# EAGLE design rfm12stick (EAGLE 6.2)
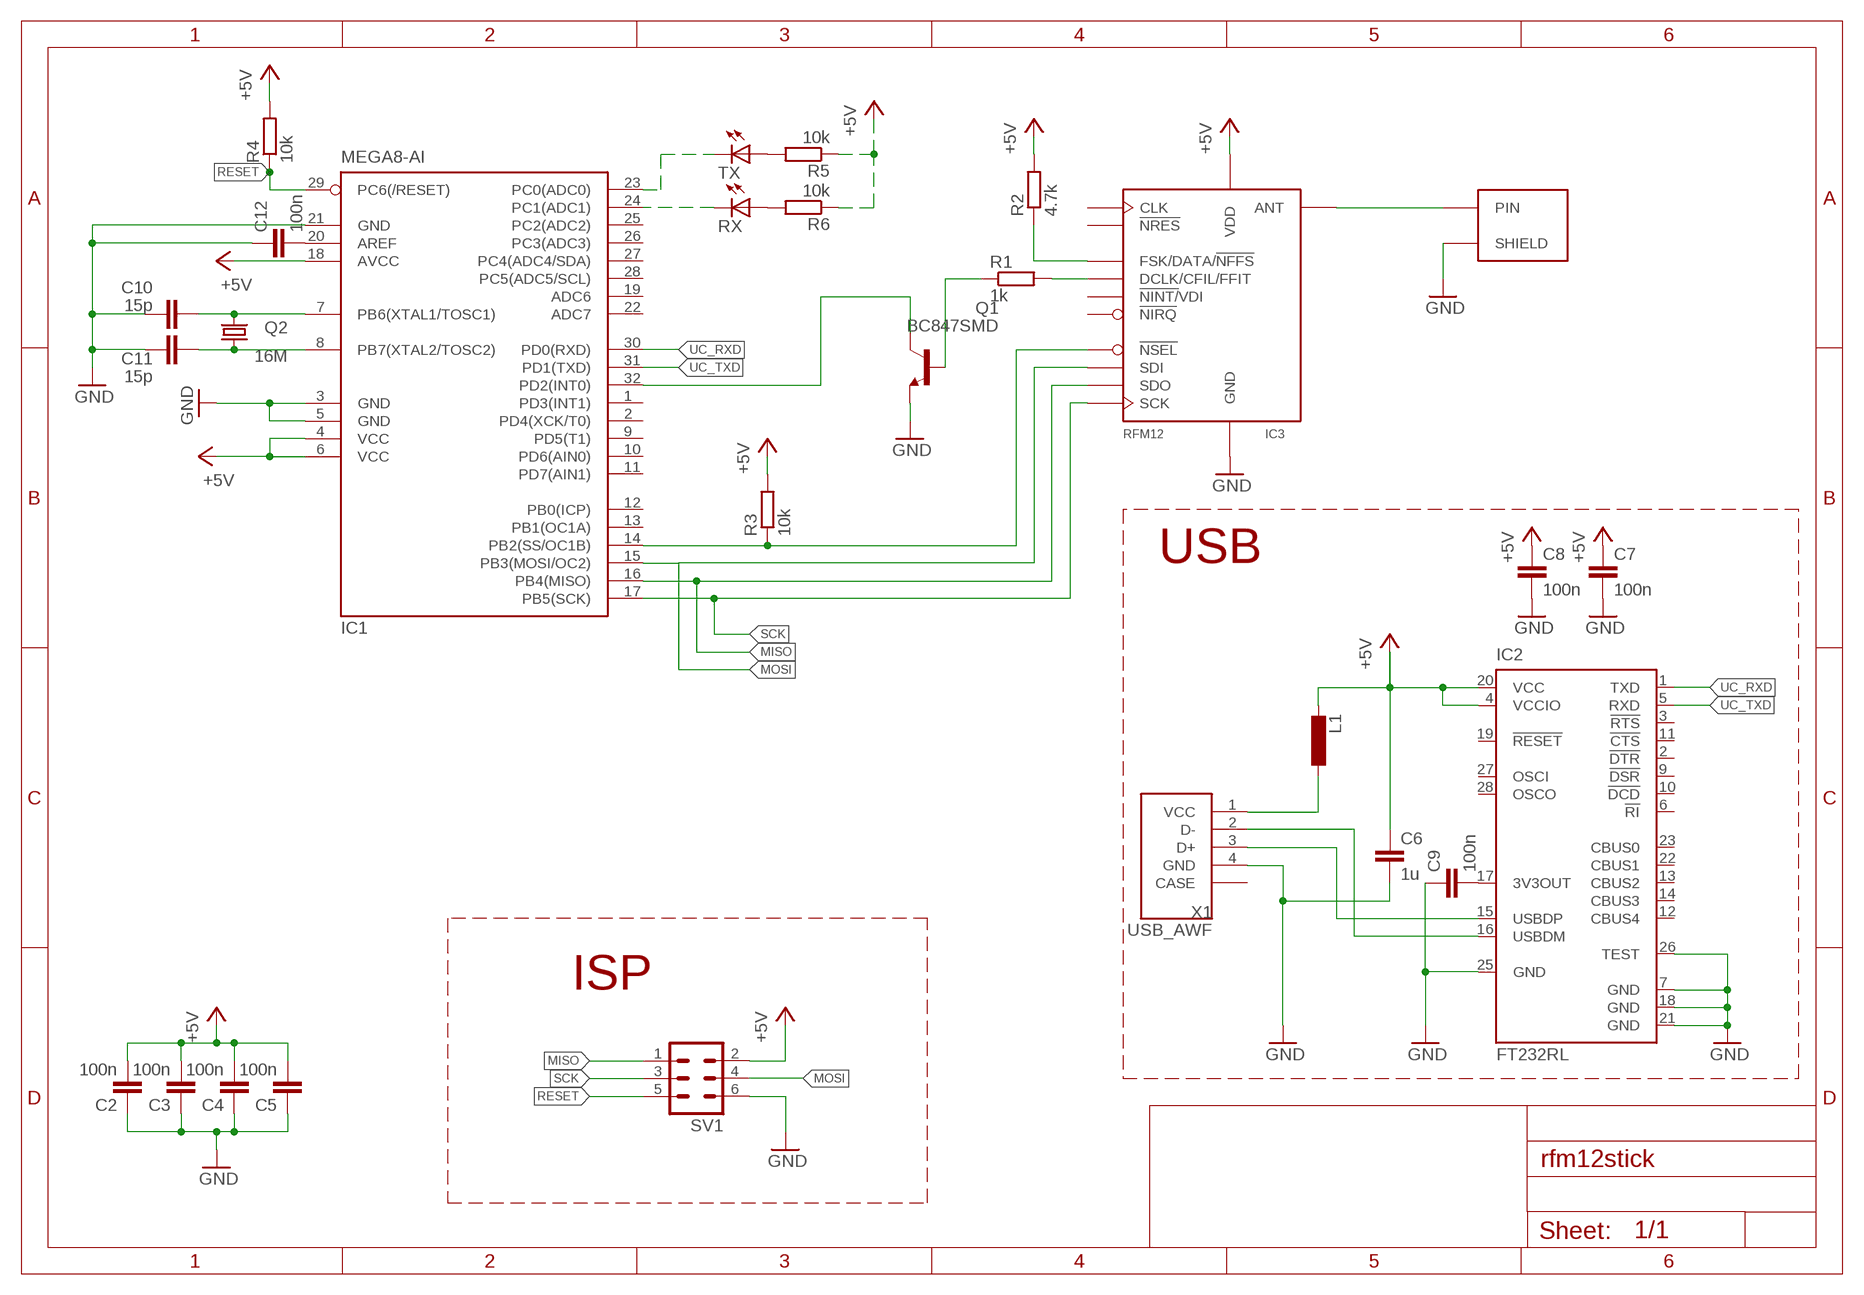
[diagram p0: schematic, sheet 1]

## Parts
C2  100n  C0805  [0805]
C3  100n  C0805  [0805]
C4  100n  C0805  [0805]
C5  100n  C0805  [0805]
C6  1u  C0805  [0805]
C7  100n  C0805  [0805]
C8  100n  C0805  [0805]
C9  100n  C0805  [0805]
C10  15p  C0805  [0805]
C11  15p  C0805  [0805]
C12  100n  C0805  [0805]
IC1  MEGA8-AI  [TQFP32-08]
IC2  FT232RL  [SSOP28]
IC3  RFM12  [RFM12_SMD_S1]
L1  L08050805  [0805]
Q1  BC847SMD  [SOT23]
Q2  16M  CRYSTALSM49  [SM49]
R1  1k  R0805  [0805]
R2  4.7k  R0805  [0805]
R3  10k  R0805  [0805]
R4  10k  R0805  [0805]
R5  10k  R0805  [0805]
R6  10k  R0805  [0805]
RX  LEDCHIPLED_0805  [CHIPLED_0805]
SV1  MA03-2  [MA03-2]
TX  LEDCHIPLED_0805  [CHIPLED_0805]
X1  USB_AWF  [USBAWF]
X2  SMA_LP_1.57MM  [SMA_LP_1.57MM]

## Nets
+5V: C2.2 C3.2 C4.2 C5.2 C6.1 C7.1 C8.1 IC1.4(VCC) IC1.6(VCC) IC1.18(AVCC) IC2.4(VCCIO) IC2.20(VCC) IC3.VDD L1.2 R2.2 R3.2 R4.2 R5.1 R6.1 SV1.2
GND: C2.1 C3.1 C4.1 C5.1 C6.2 C7.2 C8.2 C9.1 C10.1 C11.1 C12.1 IC1.3(GND) IC1.5(GND) IC1.21(GND) IC2.7(GND) IC2.18(GND) IC2.21(GND) IC2.25(GND) IC2.26(TEST) IC3.GND@1(GND) IC3.GND@2(GND) Q1.2(E) SV1.6 X1.4(GND) X2.GND(SHIELD) X2.GND@1(SHIELD) X2.GND@2(SHIELD) X2.GND@3(SHIELD)
MISO: IC1.16(PB4(MISO)) IC3.SDO SV1.1
MOSI: IC1.15(PB3(MOSI/OC2)) IC3.SDI SV1.4
N$1: IC1.14(PB2(SS/OC1B)) IC3.NSEL(!NSEL) R3.1
N$2: IC3.ANT X2.PIN
N$3: R5.2 TX.A
N$4: R6.2 RX.A
N$5: IC1.23(PC0(ADC0)) TX.C
N$6: C9.2 IC2.17(3V3OUT)
N$7: Q1.1(B) R1.1
N$8: IC3.FSK(FSK/DATA/!NFFS) R2.1
N$9: IC1.32(PD2(INT0)) Q1.3(C)
N$10: IC3.DCLK(DCLK/CFIL/FFIT) R1.2
N$11: IC1.24(PC1(ADC1)) RX.C
N$12: C10.2 IC1.7(PB6(XTAL1/TOSC1)) Q2.2
N$13: C11.2 IC1.8(PB7(XTAL2/TOSC2)) Q2.1
N$14: L1.1 X1.1(VCC)
N$17: IC2.15(USBDP) X1.3(D+)
N$18: IC2.16(USBDM) X1.2(D-)
N$19: C12.2 IC1.20(AREF)
RESET: IC1.29(PC6(/RESET)) R4.1 SV1.5
SCK: IC1.17(PB5(SCK)) IC3.SCK SV1.3
UC_RXD: IC1.30(PD0(RXD)) IC2.1(TXD)
UC_TXD: IC1.31(PD1(TXD)) IC2.5(RXD)
Unconnected: IC1.1(PD3(INT1)) IC1.2(PD4(XCK/T0)) IC1.9(PD5(T1)) IC1.10(PD6(AIN0)) IC1.11(PD7(AIN1)) IC1.12(PB0(ICP)) IC1.13(PB1(OC1A)) IC1.19(ADC6) IC1.22(ADC7) IC1.25(PC2(ADC2)) IC1.26(PC3(ADC3)) IC1.27(PC4(ADC4/SDA)) IC1.28(PC5(ADC5/SCL)) IC2.2(!DTR) IC2.3(!RTS) IC2.6(!RI) IC2.9(!DSR) IC2.10(!DCD) IC2.11(!CTS) IC2.12(CBUS4) IC2.13(CBUS2) IC2.14(CBUS3) IC2.19(!RESET) IC2.22(CBUS1) IC2.23(CBUS0) IC2.27(OSCI) IC2.28(OSCO) IC3.CLK IC3.NINT(!NINT/!VDI) IC3.NIRQ(!NIRQ) IC3.NRES(!NRES) X1.CASE X1.CASE2(CASE)

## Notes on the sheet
- USB
- ISP

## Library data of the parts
C2-C12 = R_C_0805:C0805
IC1 = atmel:MEGA8: MICROCONTROLLER 8 Kbytes FLASH, 1 kbytes SRAM, 512 bytes EEPROM, USART, 6-channel 10 bit ADC, 2-channel 8 bit ADC Pin compatible with Atmega48, ATMega88, ATMega168 Source: avr.lbr; MPN: ATMEGA8-16AU; OC_FARNELL: 9171371; OC_NEWARK: 73M8863
IC2 = ftdichip:FT232R: Source: http://www.ftdichip.com/Documents/DataSheets/DS_FT232R_v104.pdf; MPN: FT232RL; OC_FARNELL: 1146032; OC_NEWARK: 91K9918
IC3 = rf12:RFM12
L1 = R_C_0805:L0805
Q1 = transistor-npn:BC847*: NPN Transistor
Q2 = crystal:CRYSTAL: CRYSTAL; OC_FARNELL: unknown; OC_NEWARK: unknown
R1-R6 = R_C_0805:R0805
RX TX = led:LED: LED
SV1 = con-lstb:MA03-2: PIN HEADER; OC_FARNELL: unknown; OC_NEWARK: unknown
X1 = usb_awf:USB_AWF
X2 = con_sma:SMA_LP_1.57MM: Abschlussbuchse SMA LP rund 1,57mm

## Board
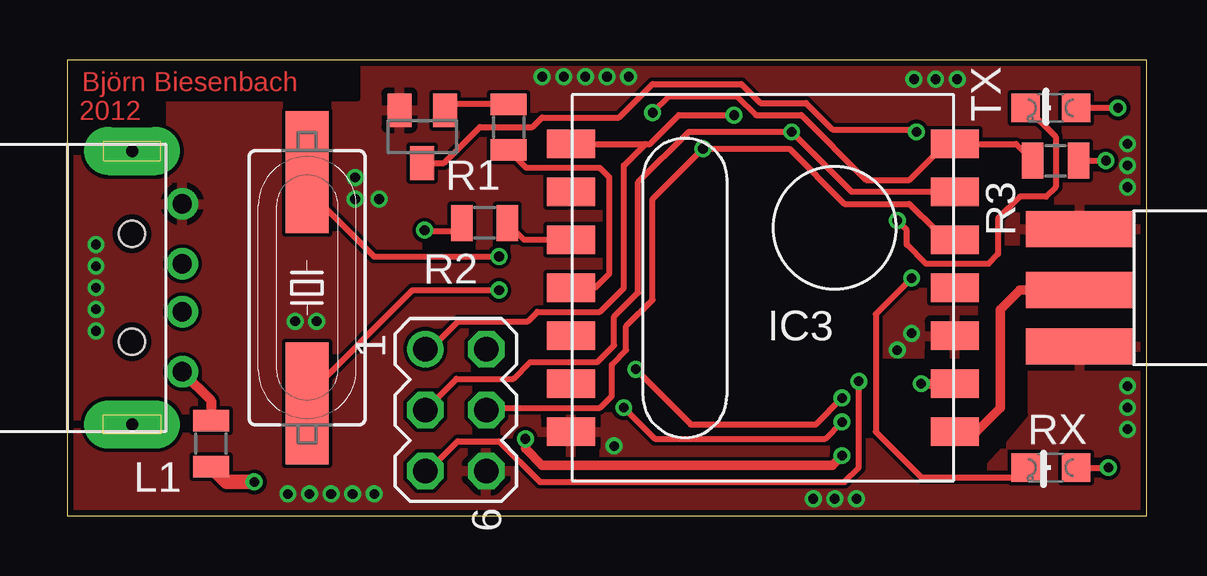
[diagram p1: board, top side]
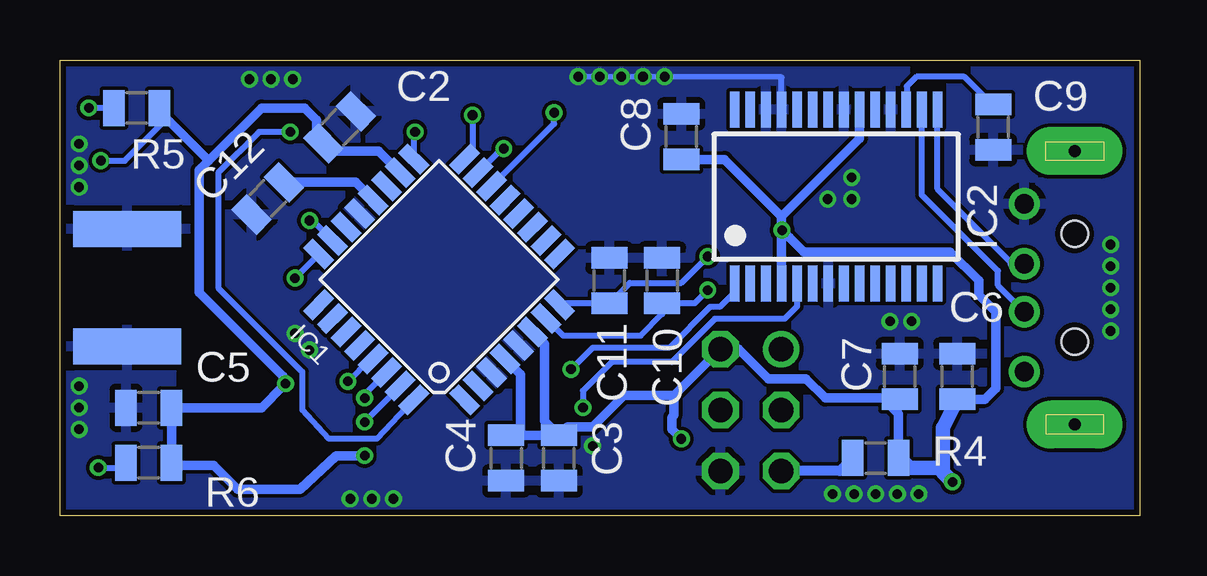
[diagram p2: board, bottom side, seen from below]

Size 45 x 19 mm. Coordinates in mm from the lower left corner, seen from the top.
Outline: 0,0 45,0 45,19 0,19 0,0
Copper layers (1*16): Top 0.035mm / dielectric 1.5mm / Bottom 0.035mm
Design rules: minimum track width 6mil, minimum drill 12mil, track to track 6mil, track to pad 6mil, pad to pad 6mil, via to via 6mil, smd to smd 0mil, copper to edge 10mil, drill to drill 10mil, minimum pad ring 10mil, minimum via ring 6mil, stop-mask expansion 2mil, vias tented up to drill 100mil, thermal gap 10mil
tRestrict: area 38.1,3 to 39.9,10.3; area 34,1.9 to 38.9,6.4; area 39.1,7.8 to 44.9,11.1; area 0.2,16.4 to 12.1,18.8
bRestrict: area 36.2,4.9 to 44.8,10.9

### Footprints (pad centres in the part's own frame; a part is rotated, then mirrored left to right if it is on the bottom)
0805 = smd 0.894 x 1.5: 1 -0.95,0; 2 0.95,0
TQFP32-08 = smd 1.27 x 0.559: 1 -4.293,2.8; 2 -4.293,2; 3 -4.293,1.2; 4 -4.293,0.4; 5 -4.293,-0.4; 6 -4.293,-1.2; 7 -4.293,-2; 8 -4.293,-2.8; 17 4.293,-2.8; 18 4.293,-2; 19 4.293,-1.2; 20 4.293,-0.4; 21 4.293,0.4; 22 4.293,1.2; 23 4.293,2; 24 4.293,2.8 | smd 0.559 x 1.27: 9 -2.8,-4.293; 10 -2,-4.293; 11 -1.2,-4.293; 12 -0.4,-4.293; 13 0.4,-4.293; 14 1.2,-4.293; 15 2,-4.293; 16 2.8,-4.293; 25 2.8,4.293; 26 2,4.293; 27 1.2,4.293; 28 0.4,4.293; 29 -0.4,4.293; 30 -1.2,4.293; 31 -2,4.293; 32 -2.8,4.293
SSOP28 = smd 0.4 x 1.5: 1 -4.225,-3.625; 2 -3.575,-3.625; 3 -2.925,-3.625; 4 -2.275,-3.625; 5 -1.625,-3.625; 6 -0.975,-3.625; 7 -0.325,-3.625; 8 0.325,-3.625; 9 0.975,-3.625; 10 1.625,-3.625; 11 2.275,-3.625; 12 2.925,-3.625; 13 3.575,-3.625; 14 4.225,-3.625; 15 4.225,3.625; 16 3.575,3.625; 17 2.925,3.625; 18 2.275,3.625; 19 1.625,3.625; 20 0.975,3.625; 21 0.325,3.625; 22 -0.325,3.625; 23 -0.975,3.625; 24 -1.625,3.625; 25 -2.275,3.625; 26 -2.925,3.625; 27 -3.575,3.625; 28 -4.225,3.625
RFM12_SMD_S1 = smd 2 x 1.2: ANT 8,-6; CLK -8,-2; DCLK -8,0; FSK -8,2; GND@1 -8,-6; GND@2 8,-2; NINT 8,0; NIRQ -8,4; NRES -8,-4; NSEL 8,6; SCK 8,4; SDI 8,2; SDO -8,6; VDD 8,-4
SOT23 = smd 1 x 1.4: 1 -0.95,-1.1; 2 0.95,-1.1; 3 0,1.1
SM49 = smd 5.08 x 1.778: 1 -4.826,0; 2 4.826,0
CHIPLED_0805 = smd 1.2 x 1.2: A 0,-1.05; C 0,1.05
MA03-2 = drill 1.016: 1 -2.54,-1.27 | drill 1.016 octagon: 2 -2.54,1.27; 3 0,-1.27; 4 0,1.27; 5 2.54,-1.27; 6 2.54,1.27
USBAWF = drill 0.8 pad 1.27: 1 3.5,10.1; 2 1,10.1; 3 -1,10.1; 4 -3.5,10.1 | drill 0.5 pad 2 long: CASE -5.7,8; CASE2 5.7,8 | hole 1.1: -2.25,8; 2.25,8
SMA_LP_1.57MM = smd 4.5 x 1.5: GND 7,2.45; GND@2 7,-2.45; PIN 7,0.1 | smd 4.5 x 1.5 bottom: GND@1 7,-2.45; GND@3 7,2.45

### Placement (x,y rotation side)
C2  33.34,16.19 225 bottom
C3  24.2,2.4 90 bottom
C4  26.4,2.4 90 bottom
C5  41.3,4.5 0 bottom
C6  7.6,5.8 90 bottom
C7  10,5.8 90 bottom
C8  19.1,15.8 90 bottom
C9  6.1,16.2 90 bottom
C10  19.9,9.8 270 bottom
C11  22.1,9.8 270 bottom
C12  36.34,13.22 45 bottom
IC1  29.2,9.85 135 bottom
IC2  12.65,13.3 0 bottom
IC3  29,9.5 0 top
L1  6,3 270 top
Q1  14.8,15.8 180 top
Q2  10,9.5 270 top
R1  18.4,16.2 270 top
R2  17.4,12.2 180 top
R3  41.2,14.8 0 top
R4  11,2.4 0 bottom
R5  41.8,17 180 bottom
R6  41.3,2.2 180 bottom
RX  41,2 90 top
SV1  16.2,4.4 270 top
TX  41,17 90 top
X1  -5.3,9.5 270 top
X2  49.2,9.5 180 top

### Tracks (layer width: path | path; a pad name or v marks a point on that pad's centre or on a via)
+5V  (via drill 0.4)
  Top 0.254: R2.2 16.45,11.85 14.95,11.85 v14.9,11.9 | R3.2 v43.3,14.8
  Top 0.4: IC3.VDD v35.6,5.5 | v19.1,3.2 19.1,2.8 19.8,2.1 31.9,2.1 v32.3,2.5
  Top 0.6: L1.2 6.65,1.4 v7.8,1.4
  Bottom 0.254: v14.9,11.9 15,11.9 15,9.75 IC2.4 | v43.3,14.8 42.3,14.8 40.55,16.55
  Bottom 0.4: R4.2 10.05,4.25 10.7,4.9 | C7.1 10.05,4.9 10.7,4.9 | IC2.4 14.93,12.47 | 14.93,12.47 11.68,15.72 IC2.20 | 19.4,5.01 SV1.2 16.71,6.94 15.47,5.7 13.9,5.7 13.1,4.9 10.7,4.9 | 19.4,5.01 19.4,4.2 19.5,4.1 19.5,3.6 v19.1,3.2 | C3.2 25.8,3.35 | 25.8,3.35 C4.2 | IC1.4 25.8,5.89 25.8,3.35 | IC1.18 31.72,15.2 33.7,15.2 C2.2 34.3,15.8 34.3,16.5 34.8,17 36.6,17 38.8,14.8 | C5.2 R6.1 40.25,2.1 38.6,2.1 37.6,1.1 35,1.1 33.5,2.5 v32.3,2.5 | C5.2 36.6,4.5 35.7,5.4 | 35.7,5.4 v35.6,5.5 | C5.2 40.35,4.75 | R5.1 40.85,16.85 40.55,16.55 38.8,14.8 | C8.1 17.3,14.85 14.93,12.47 | C6.1 6.45,4.85 6,5.3 6,8.5 6.7,9.2 6.7,9.8 7.9,11 14,11 v14.9,11.9 14.6,11.6 | IC1.6 24.8,7.15 24.8,3.95 C3.2 | 35.7,5.4 35.7,5.8 39.2,9.3 39.2,14.4 38.8,14.8 | C3.2 23.85,3.7 22.8,3.7 21.49,5.01 19.4,5.01
  Bottom 0.6: v7.8,1.4 8.2,1.8 | 8.2,1.8 8.4,2 9.6,2 10,2.4 R4.2 | C6.1 8.2,3.65 8.2,1.8
GND  (via drill 0.4)
  Bottom 0.254: IC2.25 14.93,18.27 v23.4,18.3
  other vias: 9.2,0.9 10.1,0.9 11,0.9 11.9,0.9 12.8,0.9 1.2,7.7 1.2,8.6 1.2,9.5 1.2,10.4 1.2,11.3 44.2,3.6 44.2,4.5 44.2,5.4 44.2,13.7 44.2,14.6 44.2,15.5 37.1,18.2 36.2,18.2 35.3,18.2 12,13.2 13,13.2 12,14.1 9.5,8.1 10.4,8.1 21.6,18.3 22.5,18.3 20.7,18.3 19.8,18.3 32.9,0.7 32,0.7 31.1,0.7 34.6,6.9 35.2,7.6 22.8,2.9
  pour Bottom: 0,0 45,0 45,19 0,19
  pour Top: 0,0 45,0 45,19 0,19
MISO  (via drill 0.4)
  Top 0.254: IC3.SDO 24.1,15.5 | 24.1,15.5 24.3,15.5 25.5,16.7 v27.8,16.7 | SV1.1 15.14,6.94 16.3,8.1 19.2,8.1 19.6,8.5 22.2,8.5 23.2,9.5 23.2,14.6 24.1,15.5
  Bottom 0.254: v27.8,16.7 27.8,15.2 IC1.16
MOSI  (via drill 0.4)
  Top 0.254: SV1.4 17.47,4.47 17.5,4.5 22.2,4.5 22.7,5 22.7,6.3 23.3,6.9 23.3,7.9 24.4,9 24.4,13.2 v26.5,15.3 30.1,15.3 32.4,13 35.1,13 36.2,11.9 36.6,11.9 IC3.SDI
  Bottom 0.254: IC1.15 26.57,15.3 v26.5,15.3
N$1  (via drill 0.4)
  Top 0.254: v24.4,16.8 25.1,17.5 27.9,17.5 28.7,16.7 30.6,16.7 33.3,14 35.1,14 36.6,15.5 IC3.NSEL 39.55,15.5 R3.1
  Bottom 0.254: IC1.14 24.4,16.34 v24.4,16.8
N$2
  Top 0.4: IC3.ANT 37.9,3.5 38.9,4.5 38.9,8.6 39.7,9.4 X2.PIN
N$3  (via drill 0.4)
  Top 0.254: v43.8,17 TX.A
  Bottom 0.254: R5.2 v43.8,17
N$4  (via drill 0.4)
  Top 0.254: RX.A v43.4,2
  Bottom 0.254: v43.4,2 42.45,2 R6.2
N$5  (via drill 0.4)
  Top 0.254: TX.C 40,17 41.2,15.8 41.2,13.7 40.8,13.3 39.7,13.3 38.8,12.4 38.8,10.9 38.4,10.5 35.8,10.5 35,11.3 35,11.9 v34.6,12.3
  Bottom 0.254: v34.6,12.3 34.48,12.3 IC1.23
N$6
  Bottom 0.254: C9.2 6.15,17.15 7.3,18.3 9.3,18.3 9.7,17.9 9.7,16.95 IC2.17
N$7
  Top 0.254: R1.1 16,17.15 Q1.1
N$8
  Top 0.254: IC3.FSK 19.05,11.5 R2.1
N$9  (via drill 0.4)
  Top 0.254: Q1.3 15.7,14.7 17.2,16.2 19.4,16.2 19.8,16.6 23,16.6 24.4,18 28.1,18 28.9,17.2 30.8,17.2 31.9,16.1 35.4,16.1 v35.4,16
  Bottom 0.254: v35.4,16 36.7,16 38.4,14.3 38.4,9.5 34.9,6 34.9,4.4 33.8,3.2 31.78,3.2 IC1.32
N$10
  Top 0.254: IC3.DCLK 22,9.5 22.6,10.1 22.6,14.1 22.2,14.5 19.15,14.5 R1.2
N$11  (via drill 0.4)
  Top 0.254: v35.2,9.9 33.7,8.4 33.7,3.5 35.6,1.6 39.55,1.6 RX.C
  Bottom 0.254: IC1.24 v35.2,9.9
N$12  (via drill 0.4)
  Top 0.254: 10,5 14.4,9.4 v18,9.4
  Top 0.406: Q2.2 10,5
  Bottom 0.254: 19.85,8.8 C10.2 | C10.2 19.9,8.4 20.8,7.5 24.02,7.5 IC1.7 | v18,9.4 18.55,8.85 C10.2
N$13  (via drill 0.4)
  Top 0.254: 10,13.6 12.8,10.8 v18,10.8
  Top 0.406: Q2.1 10,13.6
  Bottom 0.254: IC1.8 24.12,8.85 C11.2 21.25,9.7 19.1,9.7 v18,10.8
N$14
  Top 0.406: X1.1 6,4.8 L1.1
N$17
  Bottom 0.254: 5.3,10.5 8.43,13.62 IC2.15
  Bottom 0.4: 5.3,10.5 X1.3
N$18
  Bottom 0.254: X1.2 5.9,9.6 5.9,10.2 9.07,13.38 IC2.16
N$19
  Bottom 0.4: C12.2 32.68,13.9 IC1.20
RESET  (via drill 0.4)
  Top 0.254: SV1.5 15.04,1.86 16.28,3.1 18,3.1 19.7,1.4 32.4,1.4 33,2 v33,5.6
  Bottom 0.254: v33,5.6 32.07,6.53 IC1.29
  Bottom 0.406: R4.1 12.49,1.86 SV1.5
SCK  (via drill 0.4)
  Top 0.254: SV1.3 16.23,5.7 18.6,5.7 19.3,6.4 22.1,6.4 22.8,7.1 22.8,8.3 23.8,9.3 23.8,13.9 25.9,16 v30.2,16 32.7,13.5 IC3.SCK
  Bottom 0.254: v30.2,16 30.25,15.95 IC1.17
UC_RXD  (via drill 0.4)
  Top 0.254: v32.3,4.9 31.2,3.8 26,3.8 v23.7,6.1
  Bottom 0.254: IC2.1 16.88,9.32 17.5,8.7 17.9,8.7 19.6,7 22.8,7 v23.7,6.1 | v32.3,4.9 32.3,5.04 IC1.30
UC_TXD  (via drill 0.4)
  Top 0.254: v23.2,4.5 24.5,3.2 31.6,3.2 v32.3,3.9
  Bottom 0.254: IC2.5 14.28,8.72 14.8,8.2 17.7,8.2 19.5,6.4 22,6.4 23.2,5.2 v23.2,4.5 | v32.3,3.9 30.82,5.38 IC1.31

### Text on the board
Top: Björn Biesenbach | 2012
